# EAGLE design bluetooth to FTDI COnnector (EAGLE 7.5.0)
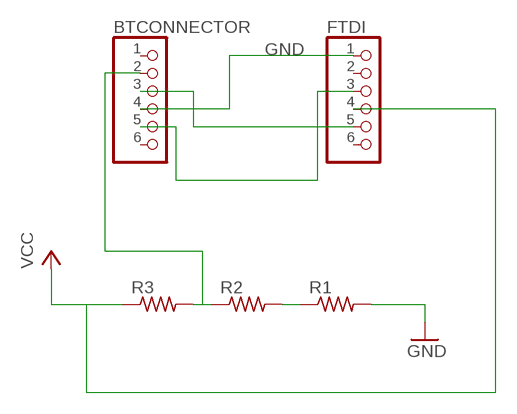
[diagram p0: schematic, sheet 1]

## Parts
BTCONNECTOR  PINHD-1X6  [1X06]
FTDI  PINHD-1X6  [1X06]
R1  RES-US1206FAB  [R1206FAB]
R2  RES-US1206FAB  [R1206FAB]
R3  RES-US1206FAB  [R1206FAB]

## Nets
GND: BTCONNECTOR.4 FTDI.1 R1.2
N$1: BTCONNECTOR.2 R2.1 R3.2
N$2: R1.1 R2.2
N$3: BTCONNECTOR.3 FTDI.5
N$4: BTCONNECTOR.5 FTDI.3
VCC: FTDI.4 R3.1
Unconnected: BTCONNECTOR.1 BTCONNECTOR.6 FTDI.2 FTDI.6

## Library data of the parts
BTCONNECTOR FTDI = pinhead:PINHD-1X6: PIN HEADER
R1-R3 = fab:RES-US: Resistor (US Symbol)

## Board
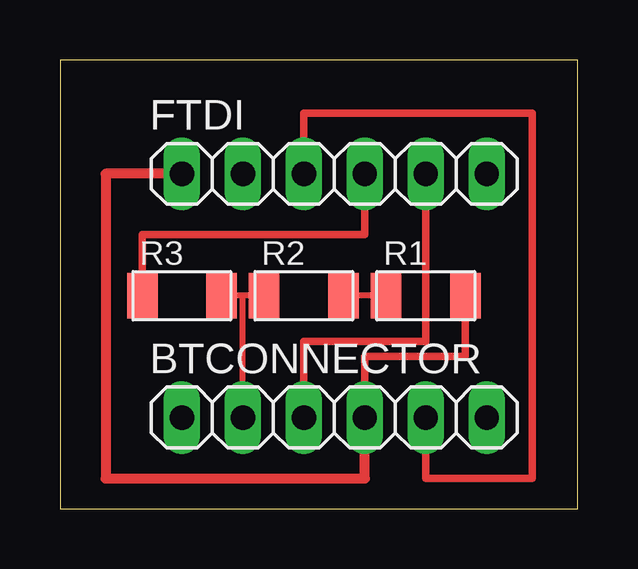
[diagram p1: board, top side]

Size 21.57 x 18.72 mm. Coordinates in mm from the lower left corner, seen from the top.
Outline: 0,0 21.57,0 21.57,18.72 0,18.72 0,0
Copper layers (1*16): Top 0.035mm / dielectric 1.5mm / Bottom 0.035mm
Design rules "default": minimum track width 10mil, minimum drill 24mil, track to track 8mil, track to pad 8mil, pad to pad 8mil, via to via 8mil, smd to smd 8mil, copper to edge 40mil, drill to drill 8mil, minimum pad ring 10mil, minimum via ring 8mil, stop-mask expansion 4mil, vias tented up to drill 0mil, thermal gap 10mil

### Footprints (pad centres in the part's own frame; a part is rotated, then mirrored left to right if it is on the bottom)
1X06 = drill 1.016 long: 1 -6.35,0; 2 -3.81,0; 3 -1.27,0; 4 1.27,0; 5 3.81,0; 6 6.35,0
R1206FAB = smd 1.27 x 1.905: 1 -1.651,0; 2 1.651,0

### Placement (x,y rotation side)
BTCONNECTOR  11.43,3.81 0 top
FTDI  11.43,13.97 0 top
R1  15.24,8.89 0 top
R2  10.16,8.89 0 top
R3  5.08,8.89 0 top

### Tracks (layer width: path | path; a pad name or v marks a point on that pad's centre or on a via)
GND
  Top 0.305: BTCONNECTOR.4 12.7,6.35 16.89,6.35 R1.2
  Top 0.406: FTDI.1 1.91,13.97 1.91,1.27 12.7,1.27 BTCONNECTOR.4
N$1
  Top 0.254: R2.1 7.62,8.89 | 7.62,8.89 R3.2 | BTCONNECTOR.2 7.62,8.89
N$2
  Top 0.254: R1.1 R2.2
N$3
  Top 0.305: FTDI.5 15.24,6.99 10.16,6.99 BTCONNECTOR.3
N$4
  Top 0.305: FTDI.3 10.16,16.51 19.68,16.51 19.68,1.27 15.24,1.27 BTCONNECTOR.5
VCC
  Top 0.305: FTDI.4 12.7,11.43 3.43,11.43 R3.1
